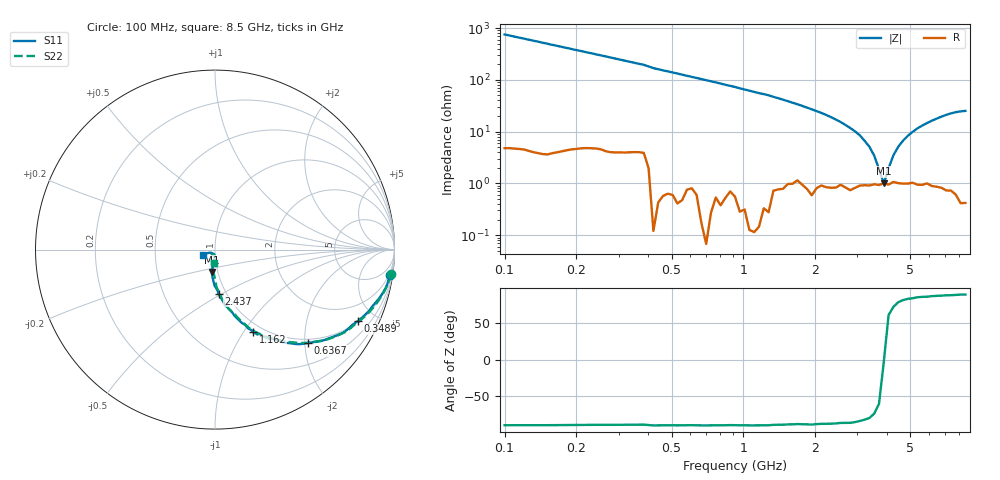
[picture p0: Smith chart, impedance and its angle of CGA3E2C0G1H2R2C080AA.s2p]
! S-parameter Generated by TDK Corporation
! Copyright(C) 2015 TDK Corporation.
! All Rights Reserved.
! TDK P/N: CGA3E2C0G1H2R2C080AA (Multilayer Ceramic Chip Capacitors)
! Property: C=2.2pF
! Size(LxWxT): 1.6x0.8x0.8mm, 0.063x0.031x0.031inches
! Model Type: s2p (Touchstone File Format Version 1.0)
! Frequency: DC=Yes Start=100MHz Stop=8500MHz 98points Log-sweep
! Note:
! Model Generated on Jun. 23, 2015
! Hash(MD5):
! Port Assignments:
!  1 ---| |--- 2
! Applicable Conditions:
!  Temperature = 25 degC
!  DC Bias Voltage = 0 V
!  Small Signal Operation
! Terms and conditions regarding TDK Simulation Models
! (1)This simulation model is being provided solely for informational purposes. Please refer to the specifications of the products in terms of detailed characteristics of such products.
! (2)In no event shall TDK Corporation of any of its subsidiaries be liable for any loss or damage arising, directly or indirectly,
!  From any information contained in this simulation model, including, but not limited to loss or damages arising from any inaccuracies, omissions or errors in connection with such information.
! (3)Any and all copyrights on this simulation model are owned by TDK Corporation.
!  Duplication or redistribution of this simulation model without prior written permission from TDK Corporation is prohibited.
! (4)This simulation model is subject to any modification or change without any prior notice.
! (5)Neither TDK Corporation nor any of its subsidiaries shall make any warranty, express or implied,
!  Including but not limited to the correctness, implied warranties of merchantability and fitness for a particular purpose with respect to this simulation models.
! (6)The use of this simulation model shall be deemed to have consented to the terms and conditions hereof.
# MHz S MA R 50
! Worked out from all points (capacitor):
!   97 points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, 100 MHz to 8.5 GHz, reference 50 ohm
!   read as one part in series: C = 2.11 pF near 100 MHz
!   lowest |Z| = 1 ohm at 3.87 GHz (marker M1)
!   series resonance near 3.876 GHz, so ESL is about 800 pH
!   S11 on the Smith chart (normalised r, x): 100 MHz: 1, -14; 348.9 MHz: 1.04, -3.96; 636.7 MHz: 0.92, -2.07; 1.162 GHz: 0.89, -1.11; 2.437 GHz: 0.92, -0.48; 8.5 GHz: 0.87, -0.05
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100  0.9858 -8.2  0.1314 81.6  0.1311 81.8  0.9899 -7.9
144.8055  0.9781 -11.6  0.1883 78.1  0.1879 78.3  0.9803 -11.4
200.2035  0.9566 -16.1  0.2554 73.5  0.2548 73.8  0.9635 -15.5
348.8583  0.8891 -26.7  0.416 62.7  0.4151 63.0  0.9001 -25.9
439.683  0.8409 -34.0  0.5222 56.4  0.5211 56.6  0.8502 -33.2
636.6849  0.7334 -45.2  0.6637 45.2  0.6624 45.5  0.7401 -44.3
840.4526  0.6364 -54.1  0.7641 36.3  0.7626 36.5  0.6379 -53.0
1161.984  0.5077 -65.1  0.8527 26.0  0.8509 26.3  0.5128 -63.8
1533.871  0.4013 -72.3  0.9034 17.5  0.9014 17.7  0.3998 -71.5
2436.519  0.2456 -85.4  0.9576 4.6  0.9552 4.8  0.2479 -83.8
2931.989  0.1939 -91.3  0.9673 -0.3  0.9651 0.1  0.2007 -88.1
3870.357  0.1254 -97.1  0.9774 -7.5  0.9747 -7.1  0.127 -93.9
4446.777  0.09047 -97.6  0.9797 -11.4  0.9787 -11.0  0.09516 -99.5
5351.035  0.06147 -88.8  0.9837 -17.1  0.9804 -16.5  0.0602 -116.4
5869.945  0.05264 -84.3  0.9842 -20.1  0.9808 -19.8  0.05109 -123.3
6147.976  0.04474 -83.9  0.9826 -21.8  0.9824 -21.3  0.04779 -127.3
6439.175  0.03891 -86.9  0.985 -23.4  0.9816 -23.0  0.0409 -126.7
7063.606  0.0247 -109.3  0.9848 -26.8  0.9818 -26.5  0.02861 -117.8
7398.175  0.02586 -130.7  0.9846 -28.7  0.9821 -28.3  0.02982 -101.9
7748.59  0.03168 -148.9  0.9844 -30.8  0.9815 -30.0  0.0368 -93.1
8115.603  0.05127 -156.0  0.9836 -32.7  0.9833 -32.1  0.05322 -94.9
8500  0.07465 -157.2  0.9815 -34.9  0.9801 -34.2  0.07543 -95.9
